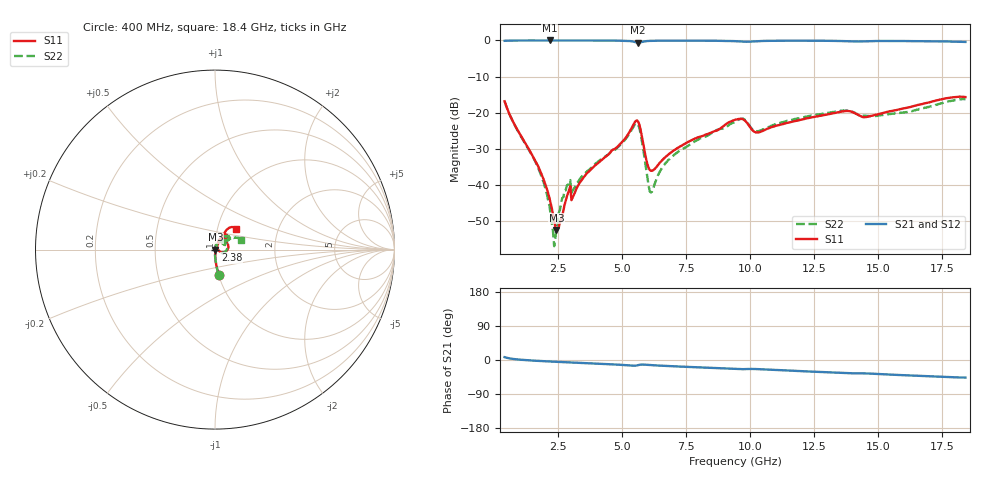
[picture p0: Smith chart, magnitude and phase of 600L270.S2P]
!  American Technical Ceramics  Date:  10/27/06
!  One Norden Lane
!  Huntington Station,  NY.  11746-2102
!  Tel:  (631) 622-4700  Fax:  (631) 622-4748
!  Part Number  600L270		Mounting Orientation: Vertical
!  Description: Ultra Low ESR Microwave capacitors
!  Application: Coupling, Bypass, Tuning, DC Block
!  Filters, Matching
# GHZ S DB R 50
! Freq  |S11|  S11 Ph  |S21|  S21 Ph  |S12|  S12 Ph  |S22|  S22 Ph
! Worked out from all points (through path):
!   401 points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, 400 MHz to 18.4 GHz, reference 50 ohm
!   highest |S21| = -0.01 dB at 2.155 GHz (marker M1); lowest = -0.6 dB at 5.62 GHz (marker M2)
!   group delay of S21, straight-line fit = 7.33 ps
!   lowest |S11| = -52.5 dB at 2.425 GHz (marker M3), VSWR 1.00, Z = 50.2 - j0.0451 ohm
!   |S11| at or under -10 dB: start of sweep to end of sweep
!   |S22| runs from -57.0 to -16.2 dB; largest |S21 - S12| = 0.0013
!   S11 on the Smith chart (normalised r, x): 400 MHz: 1.00, -0.29; 2.38 GHz: 1.00, -0.00; 18.4 GHz: 1.23, +0.29
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0.4  -16.86 -81.7  -0.11 7.5  -0.11 7.5  -16.82 -81.5
1.705  -34.77 -86.1  -0.01 -2.3  -0.01 -2.3  -35.18 -91.4
1.975  -39.55 -80.5  -0.01 -3.3  -0.01 -3.3  -40.61 -87.6
2.155  -43.77 -71.6  -0.01 -3.9  -0.01 -3.9  -45.84 -81.0
2.29  -48.14 -55.2  -0.01 -4.4  -0.01 -4.4  -52.87 -50.0
2.38  -51.51 -29.4  -0.01 -4.7  -0.01 -4.7  -54.92 1.2
2.425  -52.53 -11.0  -0.01 -4.8  -0.01 -4.8  -52.16 36.5
2.605  -49.51 50.3  -0.02 -5.4  -0.02 -5.4  -45.04 52.7
2.83  -43.28 86.1  -0.02 -6.1  -0.02 -6.1  -40.19 53.0
3.1  -42.87 68.3  -0.02 -6.9  -0.02 -6.9  -41.12 82.6
3.415  -38.66 73.0  -0.02 -7.8  -0.02 -7.8  -37.68 80.2
5.62  -22.51 7.3  -0.64 -13.5  -0.64 -13.5  -23.35 3.8
6.07  -35.88 6.9  -0.13 -13.2  -0.13 -13.2  -41.81 0.6
6.16  -36.11 22.2  -0.10 -13.7  -0.10 -13.6  -41.87 33.2
6.43  -34.17 48.4  -0.07 -14.7  -0.07 -14.7  -36.78 65.3
7.195  -29.63 62.0  -0.05 -17.2  -0.05 -17.2  -30.78 69.3
9.4  -21.99 53.0  -0.20 -23.6  -0.20 -23.6  -22.48 44.9
9.715  -21.85 39.1  -0.33 -24.2  -0.33 -24.2  -21.67 32.2
10.3  -25.50 43.9  -0.19 -24.1  -0.19 -24.1  -25.18 38.4
12.415  -21.31 57.1  -0.08 -30.7  -0.08 -30.7  -20.81 52.5
15.43  -19.62 60.1  -0.15 -38.4  -0.15 -38.4  -20.35 37.6
18.4  -15.68 43.8  -0.42 -46.4  -0.41 -46.4  -16.26 20.4
